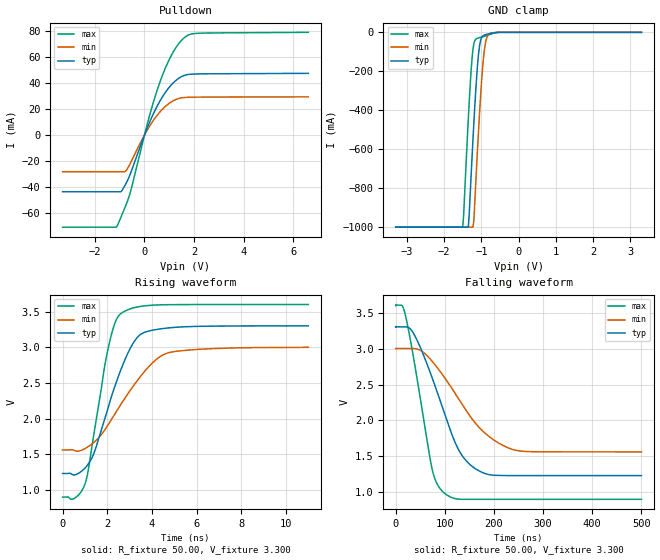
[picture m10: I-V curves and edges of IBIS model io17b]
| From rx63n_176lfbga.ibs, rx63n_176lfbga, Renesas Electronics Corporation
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[Model]   io17b
Model_type   I/O_open_drain
Polarity   Non-Inverting
Enable   Active-High
Vinl  =   0.990V
Vinh  =   2.310V
Vmeas =   1.650V
Rref  =   882.000
Cref  =   30.00pF
Vref  =   3.300V
| variable   typ   min   max
C_comp   5.360pF   5.360pF   5.360pF
| variable   typ   min   max
[Temperature Range]   45.000   105.000   -40.000
| variable   typ   min   max
[Voltage Range]   3.300V   3.000V   3.600V
| variable   typ   min   max
[Pulldown Reference]   0.000V   0.000V   0.000V
| variable   typ   min   max
[POWER Clamp Reference] 3.300V   3.000V   3.600V
| variable   typ   min   max
[GND Clamp Reference]   0.000V   0.000V   0.000V
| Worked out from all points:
|   slope of the pulldown table from 0 to 0.495 V, typ, clamps not added: 22.9 ohm
|   GND clamp passes 1 mA (typ) near -0.60 V on its own axis
|   rising waveform, R_fixture 50.00, V_fixture 3.300: 20-80 % time 1.33ns typ, 1.91ns min, 863ps max; typ from 1.23 V to 3.3 V
|   falling waveform, R_fixture 50.00, V_fixture 3.300: 20-80 % time 66.1ns typ, 90.4ns min, 39.2ns max; typ from 3.3 V to 1.23 V
[Pulldown]
| io17b_strong Pulldown rx631_rx63n
| Thu Mar 22 17:15:49 2012
| voltage   I(typ)   I(min)   I(max)
-3.3V     -43.48mA   -28.12mA   -70.65mA
-1.125V   -43.48mA   -28.12mA   -70.45mA
-925mV    -43.04mA   -28.12mA   -61.88mA
-725mV    -36.39mA   -26.83mA   -52.7mA
-525mV    -27.5mA    -19.93mA   -40.68mA
225mV     10.67mA    7.419mA    16.42mA
650mV     27mA       18.36mA    42.09mA
900mV     34.29mA    22.96mA    53.97mA
1.15V     39.89mA    26.22mA    63.48mA
1.625V    45.88mA    28.86mA    75.01mA
2.2V      46.92mA    29.1mA     78.1mA
6.6V      47.34mA    29.32mA    78.82mA
[GND Clamp]
| io17b_strong GNDClamp rx631_rx63n
| Thu Mar 22 17:15:49 2012
| voltage   I(typ)   I(min)   I(max)
-3.3V     -1A        -1A        -1A
-1.5V     -1A        -1A        -1A
-1.35V    -1A        -1A        -446.1mA
-1.275V   -737.9mA   -1A        -198mA
-1.225V   -551.1mA   -1A        -86.96mA
-1.2V     -462.3mA   -965.5mA   -57.28mA
-1.15V    -298.3mA   -774mA     -35.49mA
-1.05V    -71.6mA    -420.4mA   -27.37mA
-950mV    -16.75mA   -147.3mA   -22.23mA
-875mV    -11.42mA   -41.62mA   -18.1mA
-800mV    -8.025mA   -10.44mA   -13.02mA
3.3V      0A         0A         0A
[POWER Clamp]
| io17b_strong PWRClamp rx631_rx63n
| Thu Mar 22 17:15:49 2012
| voltage   I(typ)   I(min)   I(max)
-3.3V     0A         0A         0A
0V        0A         0A         0A
3.3V      0A         0A         0A
[Ramp]
dV/dt_r   1.241/1.33n   0.863/1.91n   1.620/862.27p
dV/dt_f   1.241/65.99n   0.863/90.30n   1.620/39.18n
R_load = 50.00ohm
[Rising Waveform]
| io17b_strong Rising-High rx631_rx63n
| Thu Mar 22 17:15:49 2012
R_fixture = 50.00
V_fixture = 3.300
V_fixture_min = 3.000
V_fixture_max = 3.600
C_fixture = 0.00pF
| Time   V(typ)   V(min)   V(max)
0s        1.232V     1.562V     901mV
550ps     1.212V     1.552V     888mV
1.02ns    1.314V     1.584V     1.1V
1.415ns   1.525V     1.671V     1.809V
2.015ns   2.127V     1.903V     2.949V
2.31ns    2.426V     2.051V     3.31V
2.61ns    2.686V     2.2V       3.472V
3.44ns    3.168V     2.573V     3.571V
4.7ns     3.271V     2.92V      3.597V
11ns      3.3V       3V         3.6V
[Falling Waveform]
| io17b_strong Falling-High rx631_rx63n
| Thu Mar 22 17:15:49 2012
R_fixture = 50.00
V_fixture = 3.300
V_fixture_min = 3.000
V_fixture_max = 3.600
C_fixture = 0.00pF
| Time   V(typ)   V(min)   V(max)
0s        3.3V       3V         3.6V
18.45ns   3.304V     3.003V     3.502V
38.4ns    3.188V     3.001V     2.791V
73.98ns   2.598V     2.826V     1.326V
84.15ns   2.401V     2.74V      1.118V
99.6ns    2.094V     2.596V     984mV
135ns     1.512V     2.228V     901mV
183ns     1.257V     1.816V     901mV
253.9ns   1.232V     1.574V     901mV
500ns     1.232V     1.562V     901mV
